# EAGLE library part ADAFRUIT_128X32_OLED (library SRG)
Adafriut 128x32 OLED display with I2C communication http://www.adafruit.com/products/931
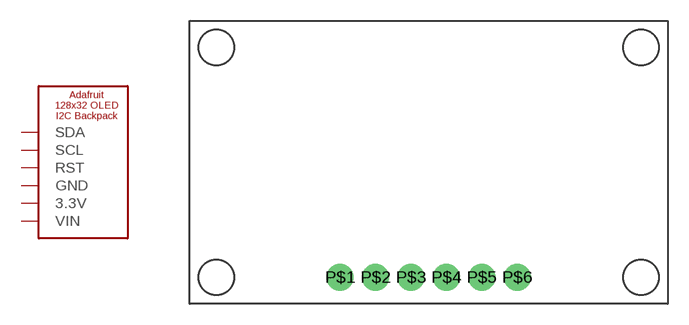
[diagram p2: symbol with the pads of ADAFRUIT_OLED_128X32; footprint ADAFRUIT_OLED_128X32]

Designator prefix -

## ADAFRUIT_128X32_OLED  [ADAFRUIT_OLED_128X32]
P$1  SDA
P$2  SCL
P$3  RST  in
P$4  GND  pwr
P$5  3.3V  pwr
P$6  VIN  pwr

## Footprint ADAFRUIT_OLED_128X32 (pad centres in mm)
128 x 32 OLED from Adafruit http://www.adafruit.com/products/931
drill 1 pad 1.93: P$1 -6.985,-6.985; P$2 -4.445,-6.985; P$3 -1.905,-6.985; P$4 0.635,-6.985; P$5 3.175,-6.985; P$6 5.715,-6.985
